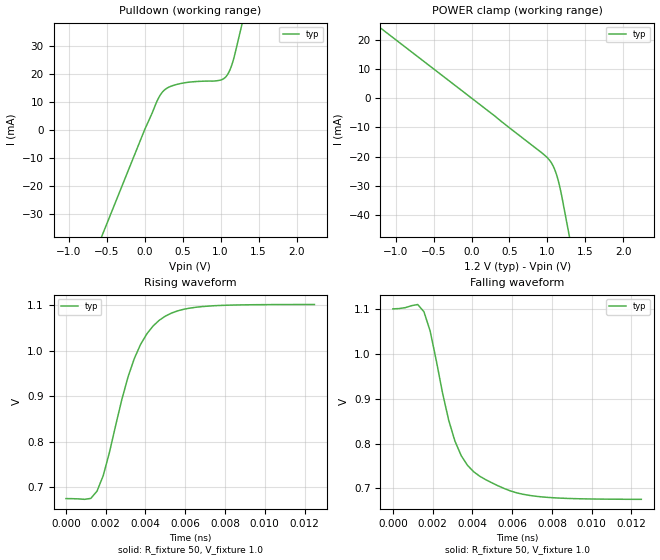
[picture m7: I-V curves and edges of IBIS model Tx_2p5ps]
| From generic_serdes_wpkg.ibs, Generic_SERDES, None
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[Model]   Tx_2p5ps
Model_type  Open_sink
C_comp 1.0p  NA  NA
Cref = 0
Vref = 0.8
Rref = 50
Vmeas = 0.8
[Temperature_Range]  25   100   0
[Voltage Range]   1.2   1.14  1.26
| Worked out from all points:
|   slope of the pulldown table from 0 to 0.18 V, typ, clamps not added: 16.1 ohm
|   falling waveform, R_fixture 50, V_fixture 1.0: 20-80 % time 1.58ps typ, NA min, NA max; typ from 1.1 V to 0.675 V
|   rising waveform, R_fixture 50, V_fixture 1.0: 20-80 % time 1.7ps typ, NA min, NA max; typ from 0.675 V to 1.1 V
[Pulldown]
-1.2V     -80.86mA   NA         NA
0V        0A         NA         NA
180mV     11.16mA    NA         NA
270mV     14.38mA    NA         NA
360mV     15.65mA    NA         NA
520mV     16.73mA    NA         NA
1.01V     17.8mA     NA         NA
1.06V     18.63mA    NA         NA
1.11V     20.57mA    NA         NA
1.16V     24.13mA    NA         NA
1.2V      28.29mA    NA         NA
2.4V      165.4mA    NA         NA
[POWER Clamp]
-1.2V     24mA       NA         NA
300mV     -6mA       NA         NA
975mV     -19.81mA   NA         NA
1.05V     -22.08mA   NA         NA
1.1V      -24.74mA   NA         NA
1.13V     -27.08mA   NA         NA
1.15V     -29mA      NA         NA
1.17V     -31.22mA   NA         NA
1.2V      -35.12mA   NA         NA
2.4V      -199.3mA   NA         NA
[Ramp]
| variable   typ   min   max
dV/dt_r   0.256/1.6994E-12   NA   NA
dV/dt_f   0.256/1.5782E-12   NA   NA
R_load = 50ohms
[Falling Waveform]
R_fixture = 50
V_fixture = 1.0
| Time   V(typ)   V(min)  V(max)
0s        1.101V     NA         NA
1.25ps    1.111V     NA         NA
1.563ps   1.095V     NA         NA
1.875ps   1.052V     NA         NA
2.5ps     913.1mV    NA         NA
3.125ps   805.2mV    NA         NA
3.437ps   773mV      NA         NA
4.062ps   737mV      NA         NA
6.875ps   683.9mV    NA         NA
12.5ps    675.1mV    NA         NA
[Rising Waveform]
R_fixture = 50
V_fixture = 1.0
| Time   V(typ)   V(min)  V(max)
0s        674.9mV    NA         NA
1.25ps    675.4mV    NA         NA
1.563ps   691.3mV    NA         NA
1.875ps   725.4mV    NA         NA
2.812ps   892.7mV    NA         NA
3.437ps   982.3mV    NA         NA
4.062ps   1.036V     NA         NA
4.687ps   1.066V     NA         NA
6.875ps   1.097V     NA         NA
12.5ps    1.101V     NA         NA
[Algorithmic Model]
Executable   Windows_VisualStudio_32   MentorTx_32.dll   MentorTx.ami
Executable   Windows_VisualStudio_64   MentorTx_64.dll   MentorTx.ami
Executable   Linux_gcc3.2.3_32   libMentorTx_32.so   MentorTx.ami
Executable   Linux_gcc3.2.3_64   libMentorTx_64.so   MentorTx.ami
[End Algorithmic Model]
